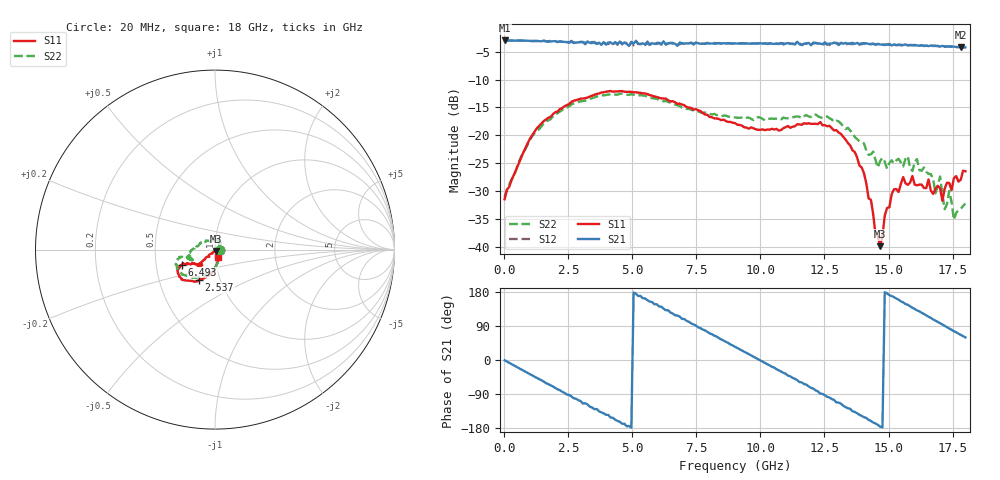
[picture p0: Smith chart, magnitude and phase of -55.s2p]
!Agilent Technologies,N5230A,US43500223,A.07.50.48
!Agilent N5230A: A.07.50.48
!Date: Sunday, January 17, 2016 17:48:57
!Correction: S11(Full 2 Port(1,2))
!S21(Full 2 Port(1,2))
!S12(Full 2 Port(1,2))
!S22(Full 2 Port(1,2))
!S2P File: Measurements: S11, S21, S12, S22:
# Hz S  dB  R 50
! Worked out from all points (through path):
!   201 points, 20 MHz to 18 GHz, reference 50 ohm
!   highest |S21| = -2.99 dB at 20 MHz (marker M1); lowest = -4.2 dB at 17.82 GHz (marker M2)
!   group delay of S21, straight-line fit = 101 ps
!   lowest |S11| = -39.8 dB at 14.67 GHz (marker M3), VSWR 1.02, Z = 50.7 - j0.752 ohm
!   |S11| at or under -10 dB: start of sweep to end of sweep
!   |S22| runs from -35.1 to -12.5 dB; largest |S21 - S12| = 0.045
!   S11 on the Smith chart (normalised r, x): 20 MHz: 1.05, -0.01; 2.537 GHz: 0.79, -0.28; 6.493 GHz: 0.68, -0.12; 18 GHz: 1.04, -0.09
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2e7  -31.43 -6.8  -2.99 -0.8  -3.00 -0.8  -30.99 -3.5
1.0988e9  -19.94 -90.0  -3.10 -40.7  -3.10 -40.9  -20.10 -88.7
2.5372e9  -14.38 -117.7  -3.38 -92.0  -3.39 -92.8  -14.80 -122.2
3.0766e9  -13.39 -124.3  -3.30 -114.8  -3.26 -113.6  -13.86 -131.5
4.515e9  -12.07 -142.2  -3.19 -163.1  -3.00 -162.6  -12.52 -153.6
6.0433e9  -13.24 -154.4  -3.45 141.5  -3.40 139.6  -13.65 -166.2
6.4928e9  -13.92 -155.3  -3.41 125.0  -3.47 124.7  -14.17 -167.5
7.9312e9  -16.31 -148.2  -3.40 74.4  -3.52 73.6  -16.08 -161.7
9.01e9  -17.80 -139.2  -3.51 34.8  -3.52 34.2  -16.79 -156.1
1.03585e10  -18.98 -130.7  -3.49 -14.1  -3.55 -15.5  -17.02 -158.4
1.20666e10  -17.92 -136.5  -3.38 -75.3  -3.58 -77.4  -16.59 -167.4
1.36848e10  -22.99 -138.4  -3.60 -136.9  -3.67 -138.9  -20.31 169.1
1.46737e10  -39.84 -46.8  -3.71 -175.7  -3.68 -176.3  -24.59 113.0
1.50333e10  -32.88 11.8  -3.62 171.1  -3.77 170.0  -24.93 95.0
1.55727e10  -27.47 8.2  -3.81 152.0  -3.88 150.2  -25.57 65.1
1.65616e10  -27.89 -14.7  -4.01 114.2  -3.93 112.2  -26.88 54.7
1.7101e10  -31.70 -36.2  -3.96 93.8  -4.07 91.7  -30.49 32.6
1.71909e10  -29.56 -36.7  -4.07 90.2  -4.13 87.6  -33.23 40.2
1.73707e10  -28.52 -53.7  -4.07 83.2  -4.07 81.0  -29.94 19.4
1.75505e10  -27.65 -49.5  -4.10 76.1  -4.15 73.9  -35.08 24.4
1.78202e10  -27.91 -57.9  -4.24 66.1  -4.23 63.8  -33.14 -23.0
1.8e10  -26.43 -65.9  -4.23 59.7  -4.25 56.9  -32.21 -10.4
